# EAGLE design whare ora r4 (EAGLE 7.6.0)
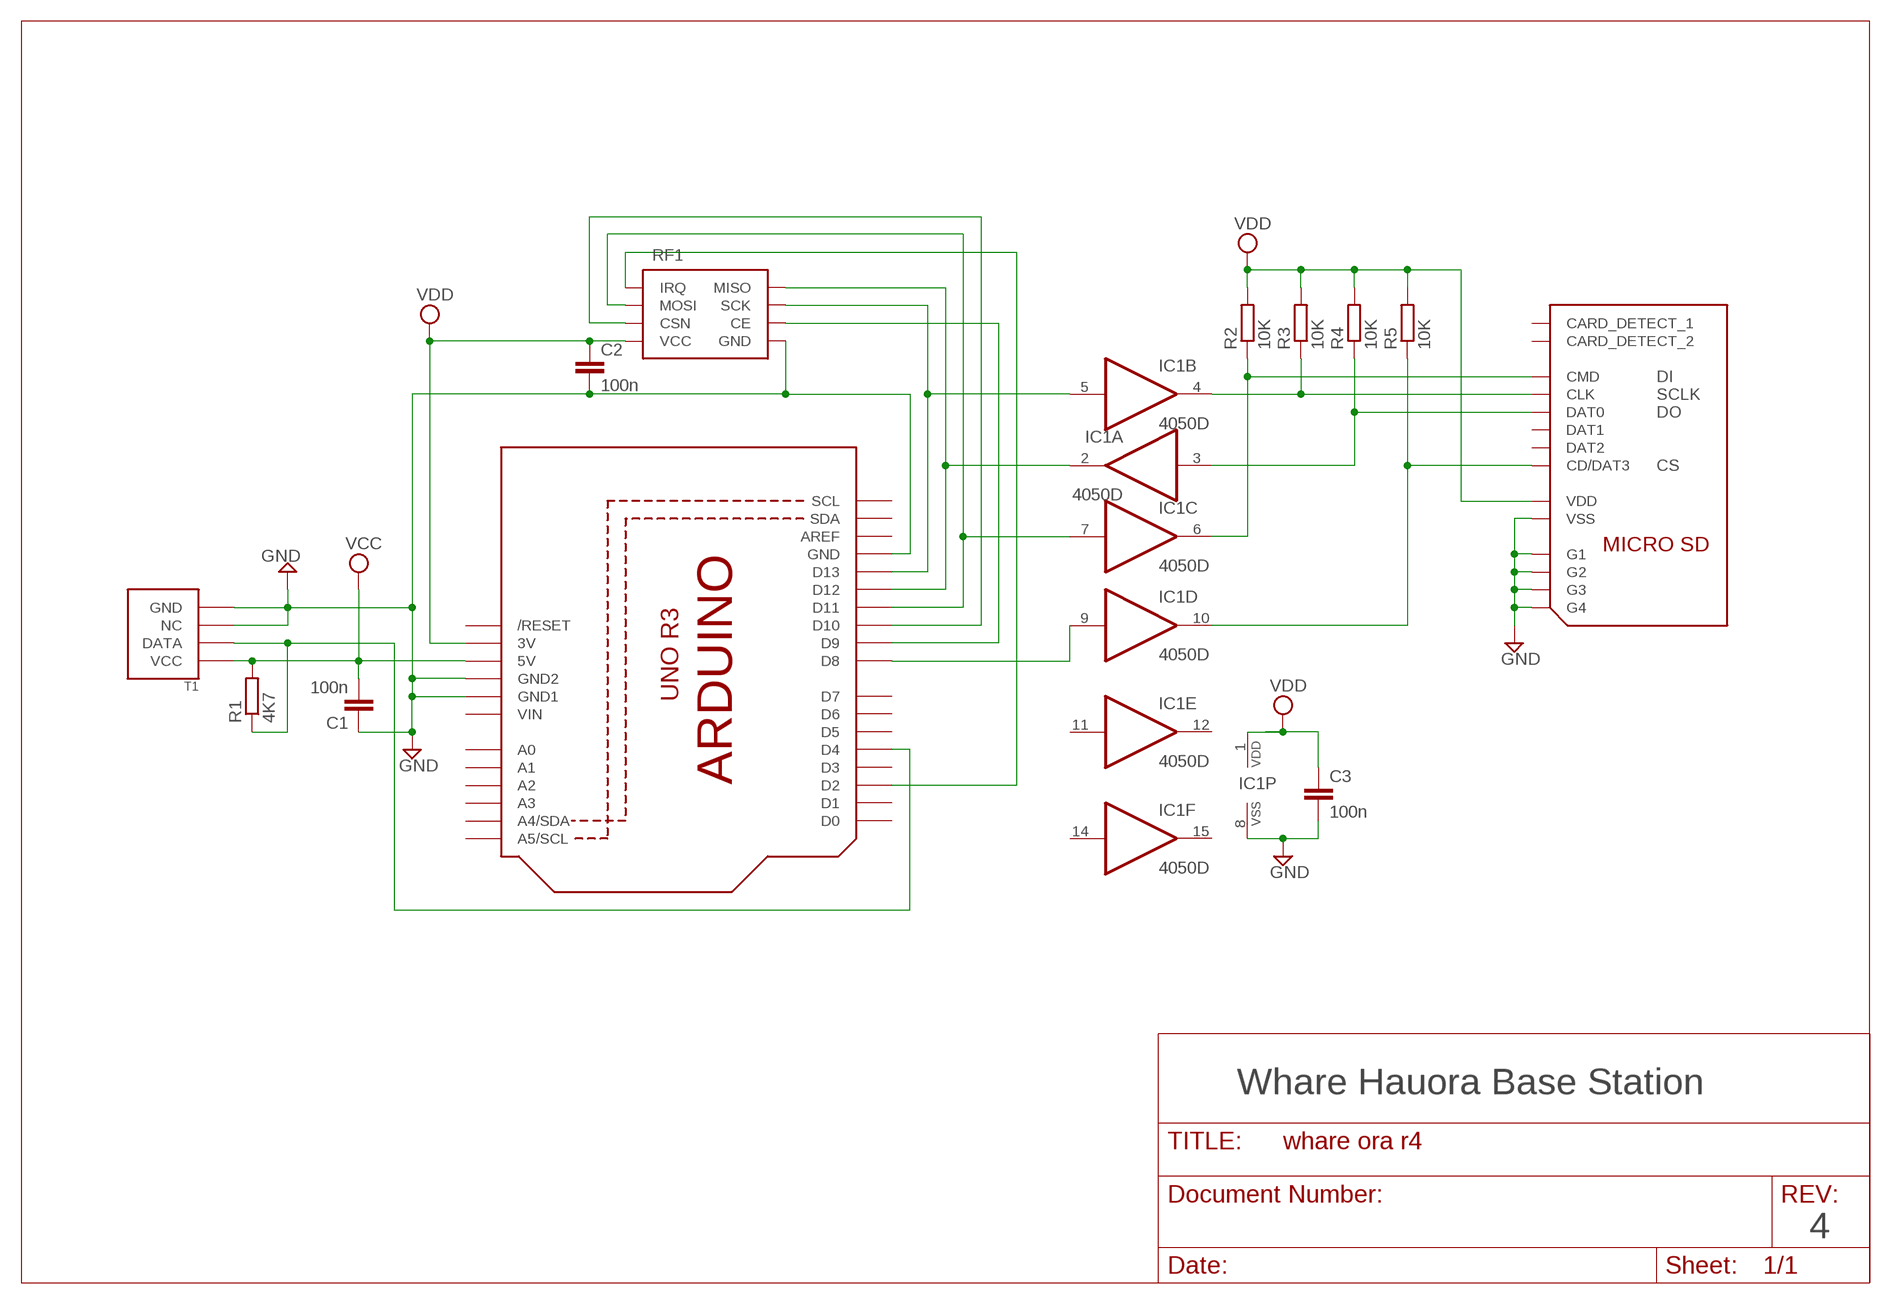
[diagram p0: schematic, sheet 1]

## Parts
C1  100n  C-EUC0805  [C0805]
C2  100n  C-EUC0805  [C0805]
C3  100n  C-EUC0805  [C0805]
IC1  4050D  [SO16]
Q1  ARDUINOR3-NOIOREFSHORT  [ARDUINOR3-NOTEXT-SHORT]
R1  4K7  R-EU_M0805  [M0805]
R2  10K  R-EU_M0805  [M0805]
R3  10K  R-EU_M0805  [M0805]
R4  10K  R-EU_M0805  [M0805]
R5  10K  R-EU_M0805  [M0805]
RF1  NRF24L01+RF2  [RF2]
SD1  MICROSD  [MICROSD]
T1  DHT22  [DHT22]

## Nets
CE: Q1.D9 RF1.P$3(CE)
CS: Q1.D10 RF1.P$4(CSN)
GND: C1.1 C2.2 C3.2 IC1.8(P:VSS) Q1.GND Q1.GND1 Q1.GND2 RF1.P$1(GND) SD1.G1 SD1.G2 SD1.G3 SD1.G4 SD1.VSS T1.P$3(NC) T1.P$4(GND)
IRQ: Q1.D2 RF1.P$8(IRQ)
MISO: IC1.2(A:O) Q1.D12 RF1.P$7(MISO)
MOSI: IC1.7(C:I) Q1.D11 RF1.P$6(MOSI)
N$2: Q1.D4 R1.1 T1.P$2(DATA)
N$5: IC1.9(D:I) Q1.D8
N$6: IC1.6(C:O) R2.1 SD1.CMD
N$7: IC1.4(B:O) R3.1 SD1.CLK
N$8: IC1.3(A:I) R4.1 SD1.DAT0
N$9: IC1.10(D:O) R5.1 SD1.CD/DAT3
SCK: IC1.5(B:I) Q1.D13 RF1.P$5(SCK)
VCC: C1.2 Q1.5V R1.2 T1.P$1(VCC)
VDD: C2.1 C3.1 IC1.1(P:VDD) Q1.3V R2.2 R3.2 R4.2 R5.2 RF1.P$2(VCC) SD1.VDD
Unconnected: IC1.11(E:I) IC1.12(E:O) IC1.14(F:I) IC1.15(F:O) Q1.A0 Q1.A1 Q1.A2 Q1.A3 Q1.A4(A4/SDA) Q1.A5(A5/SCL) Q1.AREF Q1.D0 Q1.D1 Q1.D3 Q1.D5 Q1.D6 Q1.D7 Q1.RESET(/RESET) Q1.SCL Q1.SDA SD1.CD1(CARD_DETECT_1) SD1.CD2(CARD_DETECT_2) SD1.DAT1 SD1.DAT2

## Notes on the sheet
- Whare Hauora Base Station
- 4

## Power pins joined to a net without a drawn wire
VIN: Q1.VIN

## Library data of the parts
C1-C3 = rcl:C-EU: CAPACITOR, European symbol
IC1 = 40xx:4050: Hex non-inverting BUFFER
Q1 = adafruit:ARDUINOR3-NOIOREF
R1-R5 = rcl:R-EU_: RESISTOR, European symbol
RF1 = Callum:NRF24L01+
SD1 = Callum:MICROSD
T1 = Callum:DHT

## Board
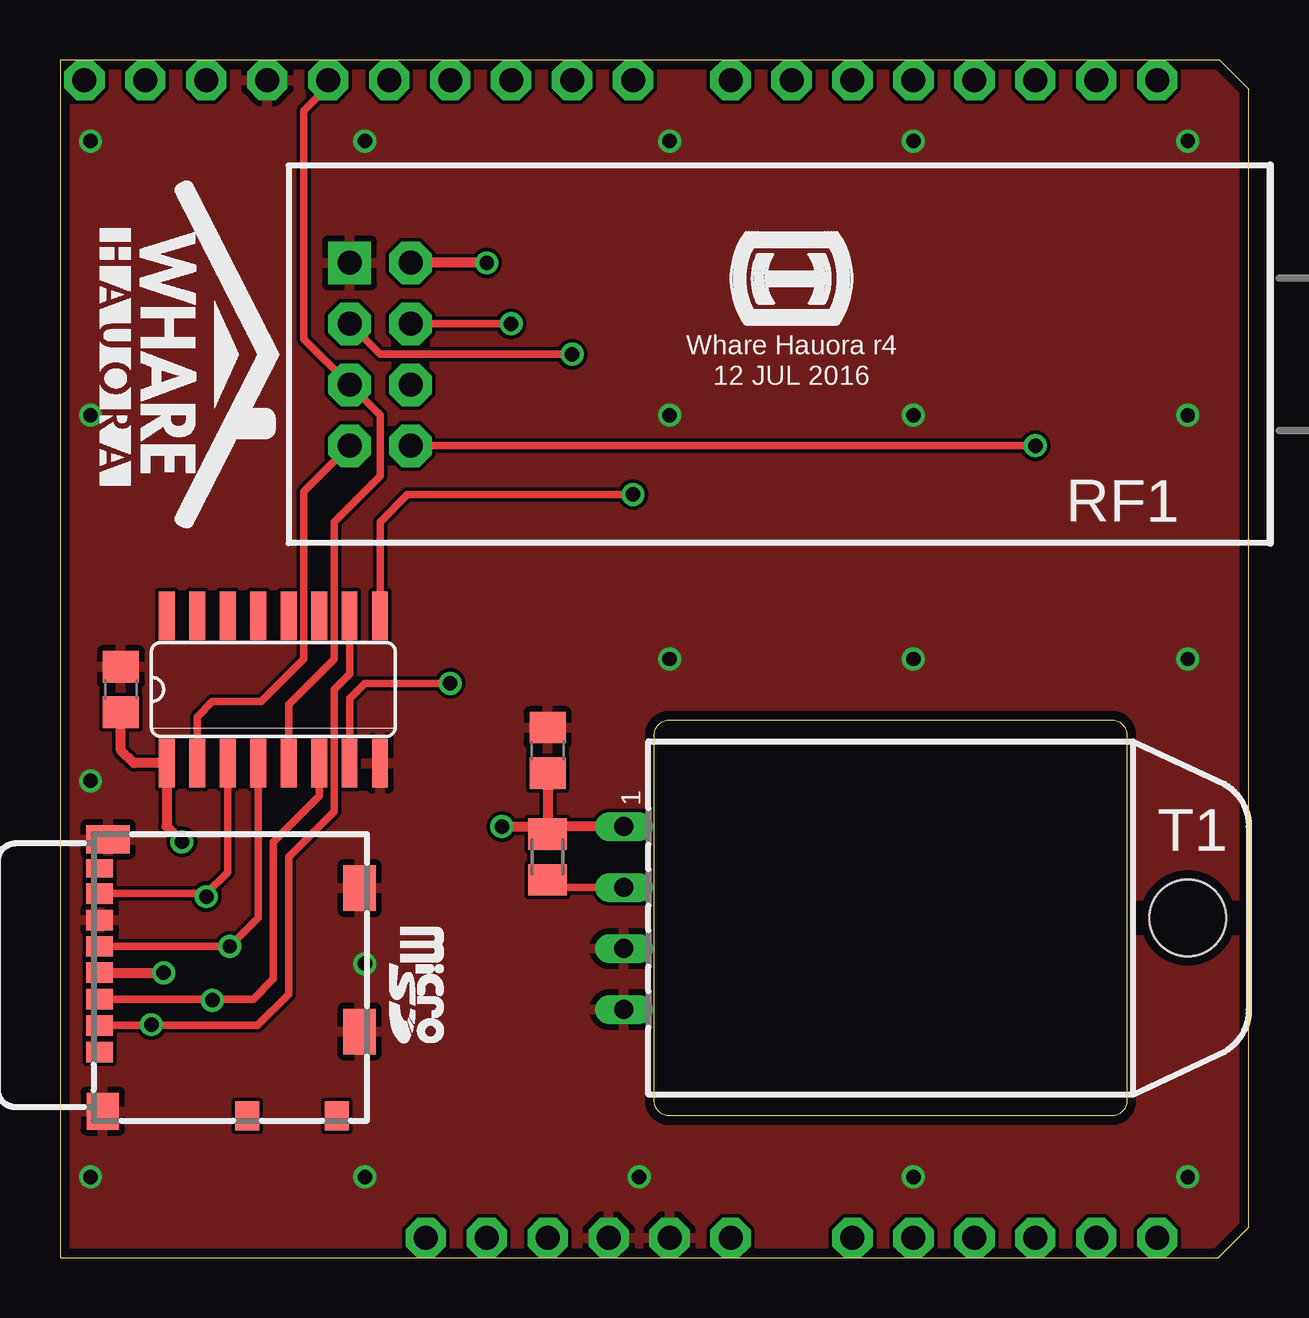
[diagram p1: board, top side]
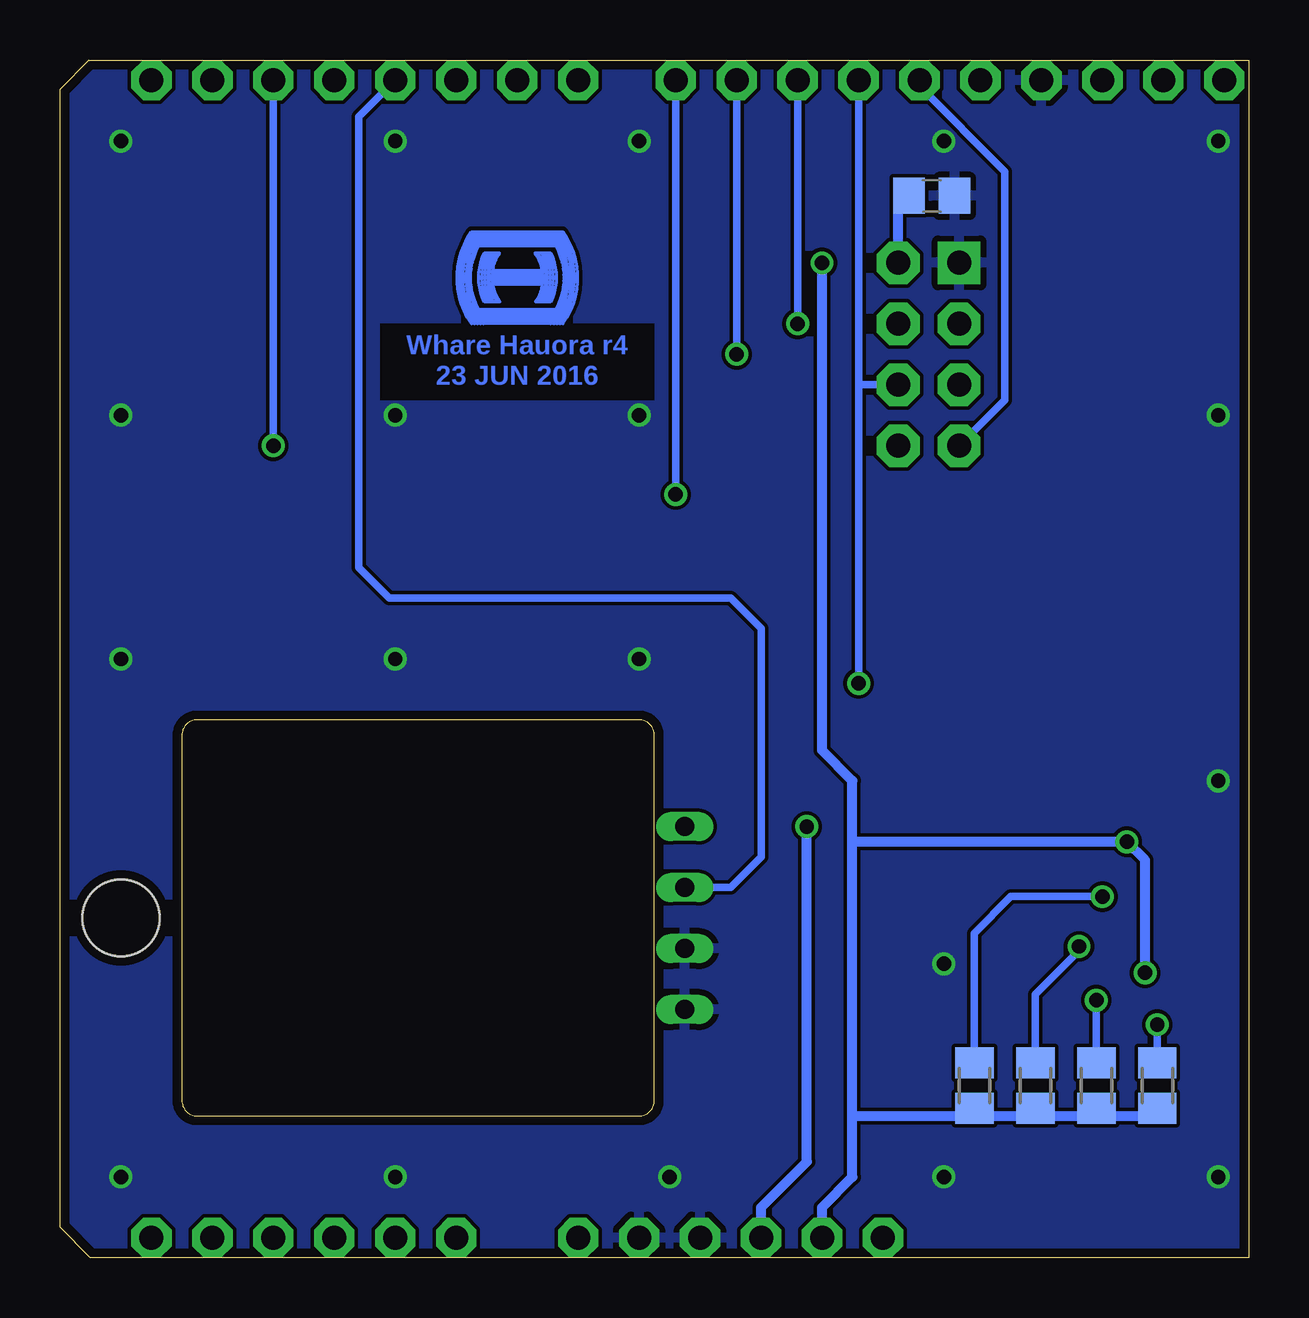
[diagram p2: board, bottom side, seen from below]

Size 49.53 x 49.91 mm. Coordinates in mm from the lower left corner, seen from the top.
Outline: 25.4,22.42 43.81,22.42 arc-90 44.45,21.78 44.45,6.54 arc-90 43.81,5.91 25.4,5.91 arc-90 24.77,6.54 24.77,21.78 arc-90 25.4,22.42
Copper layers (1*16): Top 0.0356mm / dielectric 1.5011mm / Bottom 0.0356mm
Design rules "OSHpark DRC *": minimum track width 6mil, minimum drill 13mil, track to track 6mil, track to pad 6mil, pad to pad 6mil, via to via 6mil, smd to smd 6mil, copper to edge 15mil, drill to drill 6mil, minimum pad ring 7mil, minimum via ring 7mil, stop-mask expansion 3mil, vias tented up to drill 30mil, thermal gap 10mil
bRestrict: area 24.8,35.8 to 36.2,38.9

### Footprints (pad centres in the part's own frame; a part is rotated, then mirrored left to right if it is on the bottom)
C0805 = smd 1.3 x 1.5: 1 -0.95,0; 2 0.95,0
SO16 = smd 0.66 x 2.032: 1 -4.445,-3.073; 2 -3.175,-3.073; 3 -1.905,-3.073; 4 -0.635,-3.073; 5 0.635,-3.073; 6 1.905,-3.073; 7 3.175,-3.073; 8 4.445,-3.073; 9 4.445,3.073; 10 3.175,3.073; 11 1.905,3.073; 12 0.635,3.073; 13 -0.635,3.073; 14 -1.905,3.073; 15 -3.175,3.073; 16 -4.445,3.073
ARDUINOR3-NOTEXT-SHORT = drill 1 pad 1.676 octagon: 3V 19.05,2.54; 5V 21.59,2.54; A0 34.29,2.54; A1 36.83,2.54; A2 39.37,2.54; A3 41.91,2.54; A4 44.45,2.54; A5 46.99,2.54; AREF 7.366,50.8; D0 46.99,50.8; D1 44.45,50.8; D2 41.91,50.8; D3 39.37,50.8; D4 36.83,50.8; D5 34.29,50.8; D6 31.75,50.8; D7 29.21,50.8; D8 25.146,50.8; D9 22.606,50.8; D10 20.066,50.8; D11 17.526,50.8; D12 14.986,50.8; D13 12.446,50.8; GND 9.906,50.8; GND1 26.67,2.54; GND2 24.13,2.54; RESET 16.51,2.54; SCL 2.286,50.8; SDA 4.826,50.8; VIN 29.21,2.54
M0805 = smd 1.3 x 1.6: 1 -0.95,0; 2 0.95,0
RF2 = drill 1 pad 1.778 square: P$1 0,0 | drill 1 pad 1.778 octagon: P$2 -2.54,0; P$3 0,2.54; P$4 -2.54,2.54; P$5 0,5.08; P$6 -2.54,5.08; P$7 0,7.62; P$8 -2.54,7.62
MICROSD = smd 1.2 x 1: CD1 5.704,0.826; CD2 5.704,4.536 | smd 0.85 x 1.1: CD/DAT3 1.944,-5.334; CLK -1.356,-5.334; CMD 0.844,-5.334; DAT0 -3.556,-5.334; DAT2 3.044,-5.334; VDD -0.256,-5.334; VSS -2.456,-5.334 | smd 0.75 x 1.1: DAT1 -4.606,-5.334 | smd 1.55 x 1.35: G1 5.514,-5.204 | smd 1.17 x 1.8: G2 -5.816,-4.984 | smd 1.9 x 1.35: G3 -3.786,5.496; G4 2.194,5.496
DHT22 = drill 0.8 long: P$1 0,0; P$2 2.54,0; P$3 5.08,0; P$4 7.62,0 | hole 3.2: 3.81,23.495

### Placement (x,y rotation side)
C1  20.32,21.15 270 top
C2  13.21,44.26 0 bottom
C3  2.54,23.69 90 top
IC1  8.89,23.69 0 top
Q1  -1.27,-1.71 0 top
R1  20.32,16.7 90 top
R2  6.35,7.18 270 bottom
R3  8.89,7.18 270 bottom
R4  11.43,7.18 270 bottom
R5  3.81,7.18 270 bottom
RF1  12.07,41.47 180 top
SD1  6.99,11.62 270 top
T1  23.5,17.97 270 top
U$1  [MY-LOGO-COPPER]  30.48,40.83 180 bottom
U$2  [MY-LOGO-SMALL]  30.48,40.83 0 top
U$3  [MICROSD-LOGO-SMALL]  13.72,13.78 270 top
U$5  [WHAREHAUORA-SMALL]  1.52,45.02 270 top

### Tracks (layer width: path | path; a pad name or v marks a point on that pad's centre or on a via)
CE  (via drill 0.6)
  Top 0.305: RF1.P$3 13.34,37.66 v21.34,37.66
  Bottom 0.305: Q1.D9 v21.34,37.66
CS  (via drill 0.6)
  Top 0.305: v18.8,38.93 RF1.P$4
  Bottom 0.305: Q1.D10 v18.8,38.93
GND  (via drill 0.6)
  other vias: 1.27,46.55 24.13,3.37 1.27,19.88 1.27,3.37 25.4,46.55 46.99,24.96 35.56,46.55 46.99,35.12 12.7,3.37 25.4,24.96 35.56,3.37 35.56,24.96 12.7,12.26 46.99,46.55 25.4,35.12 1.27,35.12 35.56,35.12 46.99,3.37 12.7,46.55
  pour Bottom: 0,0.19 48.26,0.19 49.53,1.46 49.53,48.45 48.26,49.72 0,49.72
  pour Top: 0,49.72 48.26,49.72 49.53,48.45 49.53,1.46 48.26,0.19 0,0.19
IRQ  (via drill 0.6)
  Top 0.305: v40.64,33.85 RF1.P$8
  Bottom 0.305: Q1.D2 v40.64,33.85
MISO
  Top 0.305: IC1.2 5.71,22.54 6.35,23.18 8.38,23.18 10.16,24.96 10.16,31.94 RF1.P$7
  Bottom 0.305: RF1.P$7 10.16,35.75 10.16,45.28 13.72,48.83 Q1.D12
MOSI  (via drill 0.6)
  Top 0.305: v16.26,23.94 12.7,23.94 12.07,23.3 IC1.7
  Bottom 0.305: Q1.D11 16.26,36.39 | 16.26,36.39 v16.26,23.94 | RF1.P$6 16.26,36.39
N$2
  Top 0.305: T1.P$2 20.64,15.43
  Top 0.406: 20.64,15.43 R1.1
  Bottom 0.305: Q1.D4 37.08,47.56 37.08,28.77 35.81,27.5 21.59,27.5 20.32,26.23 20.32,16.7 21.59,15.43 T1.P$2
N$5  (via drill 0.6)
  Top 0.305: v23.88,31.81 14.48,31.81 13.34,30.67 IC1.9
  Top 0.406: 13.34,26.73 IC1.9
  Bottom 0.305: Q1.D8 v23.88,31.81
N$6  (via drill 0.6)
  Top 0.305: IC1.6 10.79,19.24 8.89,17.34 8.89,11.62 8.05,10.78 6.35,10.78 SD1.CMD
  Top 0.406: 6.35,10.78 v6.35,10.73
  Bottom 0.305: v6.35,10.73 R2.1
N$7  (via drill 0.6)
  Top 0.305: SD1.CLK v7.07,12.98 8.26,14.16 IC1.4
  Bottom 0.305: 7.07,12.8 8.89,10.99 R3.1
  Bottom 0.406: v7.07,12.98 7.07,12.8
N$8  (via drill 0.6)
  Top 0.305: SD1.DAT0 6.1,15.18 6.99,16.07 IC1.3
  Top 0.406: 6.1,15.18 v6.1,15.05
  Bottom 0.305: v6.1,15.05 9.91,15.05 11.43,13.53 R4.1
N$9  (via drill 0.6)
  Top 0.305: IC1.10 12.07,24.32 11.43,23.69 11.43,18.61 9.53,16.7 9.53,10.99 8.22,9.68 SD1.CD/DAT3 3.77,9.68
  Top 0.406: 3.77,9.68 v3.81,9.72
  Bottom 0.305: v3.81,9.72 R5.1
SCK
  Top 0.305: Q1.D13 11.18,48.83 10.16,47.82 10.16,38.29 RF1.P$5 13.34,35.12 13.34,32.58 11.43,30.67 11.43,24.96 9.53,23.05 IC1.5
VCC  (via drill 0.6)
  Top 0.406: T1.P$1 20.32,17.97 | 20.32,17.97 20,17.97 | R1.2 20.32,17.97 | C1.2 R1.2 | v18.41,17.97 20,17.97 | 20,17.97 R1.2
  Bottom 0.406: Q1.5V 20.32,2.1 18.41,4 v18.41,17.97
VDD  (via drill 0.6)
  Top 0.406: C3.1 2.54,21.15 3.07,20.61 IC1.1 4.45,17.97 v5.08,17.34 | v17.78,41.47 RF1.P$2 | SD1.VDD v4.32,11.88 v4.32,11.87
  Bottom 0.406: 16.51,5.91 11.43,5.91 | 11.43,5.91 8.89,5.91 | 8.89,5.91 6.35,5.91 | 6.35,5.91 3.81,5.91 R5.2 | R2.2 6.35,5.91 | R3.2 8.89,5.91 | R4.2 11.43,5.91 | Q1.3V 17.78,2.1 16.51,3.37 16.51,5.91 | 16.51,5.91 16.51,17.34 | 16.51,17.34 16.51,19.88 17.78,21.15 v17.78,41.47 | v4.32,11.87 4.32,16.57 v5.08,17.34 16.51,17.34 | RF1.P$2 14.61,44.01 14.16,44.01 C2.1

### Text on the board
Bottom: Whare Hauora r4 | 23 JUN 2016
tPlace: Whare Hauora r4 | 12 JUL 2016
bValues: R2-R5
